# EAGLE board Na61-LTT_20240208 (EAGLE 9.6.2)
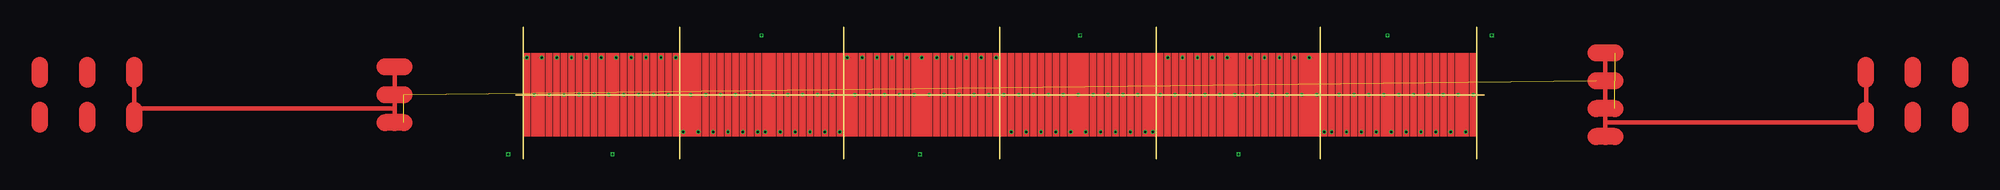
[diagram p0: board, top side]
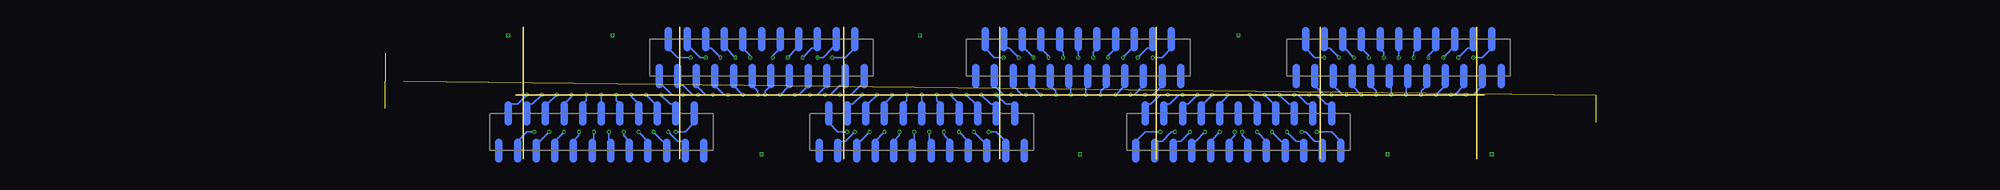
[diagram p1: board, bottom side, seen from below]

Size 104 x 14.2 mm. Coordinates in mm from the lower left corner, seen from the top.
Outline: 52,0 52,14.2
Outline: 35.2,0 35.2,14.2
Outline: 17.6,0 17.6,14.2
Outline: 0.8,0 0.8,14.2
Outline: 68.8,0 68.8,14.2
Outline: 86.4,0 86.4,14.2
Outline: 103.2,0 103.2,14.2
Outline: 0,6.9 104,6.9
Copper layers (1*16): Top 0.035mm / dielectric 1.5mm / Bottom 0.035mm
Design rules "default *": minimum track width 6mil, minimum drill 0.2mm, track to track 6mil, track to pad 6mil, pad to pad 6mil, via to via 6mil, smd to smd 6mil, copper to edge 40mil, drill to drill 6mil, minimum pad ring 8mil, minimum via ring 4mil, stop-mask expansion 4mil, vias tented up to drill 0mil, thermal gap 10mil

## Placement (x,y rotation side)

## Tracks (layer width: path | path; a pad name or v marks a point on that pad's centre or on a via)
S$1
  Bottom 0.8: 63.4,1.8 63.4,0
S$2
  Bottom 0.8: 62.4,4 62.4,5.8
S$3
  Bottom 0.8: 59.4,1.8 59.4,0
S$4
  Bottom 0.8: 56.4,4 56.4,5.8
S$5
  Bottom 0.8: 53.4,1.8 53.4,0
S$6
  Bottom 0.8: 52.4,4 52.4,5.8
S$7
  Bottom 0.8: 49.4,1.8 49.4,0
S$8
  Bottom 0.8: 50.4,4 50.4,5.8
S$9
  Bottom 0.8: 71.4,1.8 71.4,0
S$10
  Bottom 0.8: 70.4,4 70.4,5.8
S$11
  Bottom 0.8: 67.4,1.8 67.4,0
S$12
  Bottom 0.8: 66.4,4 66.4,5.8
S$13
  Bottom 0.8: 68.4,4 68.4,5.8
S$14
  Bottom 0.8: 69.4,1.8 69.4,0
S$15
  Bottom 0.8: 65.4,1.8 65.4,0
S$16
  Bottom 0.8: 64.4,4 64.4,5.8
S$17
  Bottom 0.8: 60.4,4 60.4,5.8
S$18
  Bottom 0.8: 61.4,1.8 61.4,0
S$19
  Bottom 0.8: 57.4,1.8 57.4,0
S$20
  Bottom 0.8: 58.4,4 58.4,5.8
S$21
  Bottom 0.8: 54.4,4 54.4,5.8
S$22
  Bottom 0.8: 55.4,1.8 55.4,0
S$23
  Bottom 0.8: 51.4,1.8 51.4,0
S$24
  Bottom 0.8: 44.6,9.8 44.6,8
S$25
  Bottom 0.8: 46.6,9.8 46.6,8
S$26
  Bottom 0.8: 43.6,12 43.6,13.8
S$27
  Bottom 0.8: 45.6,12 45.6,13.8
S$28
  Bottom 0.8: 40.6,9.8 40.6,8
S$29
  Bottom 0.8: 42.6,9.8 42.6,8
S$30
  Bottom 0.8: 41.6,12 41.6,13.8
S$31
  Bottom 0.8: 39.6,12 39.6,13.8
S$32
  Bottom 0.8: 38.6,9.8 38.6,8
S$33
  Bottom 0.8: 36.6,9.8 36.6,8
S$34
  Bottom 0.8: 37.6,12 37.6,13.8
S$35
  Bottom 0.8: 35.6,12 35.6,13.8
S$36
  Bottom 0.8: 34.6,9.8 34.6,8
S$37
  Bottom 0.8: 32.6,9.8 32.6,8
S$38
  Bottom 0.8: 33.6,12 33.6,13.8
S$39
  Bottom 0.8: 52.6,9.8 52.6,8
S$40
  Bottom 0.8: 54.6,9.8 54.6,8
S$41
  Bottom 0.8: 51.6,12 51.6,13.8
S$42
  Bottom 0.8: 53.6,12 53.6,13.8
S$43
  Bottom 0.8: 48.6,9.8 48.6,8
S$44
  Bottom 0.8: 50.6,9.8 50.6,8
S$45
  Bottom 0.8: 47.6,12 47.6,13.8
S$46
  Bottom 0.8: 49.6,12 49.6,13.8
S$47
  Bottom 0.8: 27.4,1.8 27.4,0
S$48
  Bottom 0.8: 29.4,1.8 29.4,0
S$49
  Bottom 0.8: 26.4,4 26.4,5.8
S$50
  Bottom 0.8: 28.4,4 28.4,5.8
S$51
  Bottom 0.8: 23.4,1.8 23.4,0
S$52
  Bottom 0.8: 25.4,1.8 25.4,0
S$53
  Bottom 0.8: 24.4,4 24.4,5.8
S$54
  Bottom 0.8: 22.4,4 22.4,5.8
S$55
  Bottom 0.8: 21.4,1.8 21.4,0
S$56
  Bottom 0.8: 19.4,1.8 19.4,0
S$57
  Bottom 0.8: 20.4,4 20.4,5.8
S$58
  Bottom 0.8: 18.4,4 18.4,5.8
S$59
  Bottom 0.8: 17.4,1.8 17.4,0
S$60
  Bottom 0.8: 15.4,1.8 15.4,0
S$61
  Bottom 0.8: 16.4,4 16.4,5.8
S$62
  Bottom 0.8: 35.4,1.8 35.4,0
S$63
  Bottom 0.8: 37.4,1.8 37.4,0
S$64
  Bottom 0.8: 34.4,4 34.4,5.8
S$65
  Bottom 0.8: 36.4,4 36.4,5.8
S$66
  Bottom 0.8: 31.4,1.8 31.4,0
S$67
  Bottom 0.8: 33.4,1.8 33.4,0
S$68
  Bottom 0.8: 30.4,4 30.4,5.8
S$69
  Bottom 0.8: 32.4,4 32.4,5.8
S$70
  Bottom 0.8: 78.6,9.8 78.6,8
S$71
  Bottom 0.8: 80.6,9.8 80.6,8
S$72
  Bottom 0.8: 77.6,12 77.6,13.8
S$73
  Bottom 0.8: 79.6,12 79.6,13.8
S$74
  Bottom 0.8: 74.6,9.8 74.6,8
S$75
  Bottom 0.8: 76.6,9.8 76.6,8
S$76
  Bottom 0.8: 75.6,12 75.6,13.8
S$77
  Bottom 0.8: 73.6,12 73.6,13.8
S$78
  Bottom 0.8: 72.6,9.8 72.6,8
S$79
  Bottom 0.8: 70.6,9.8 70.6,8
S$80
  Bottom 0.8: 71.6,12 71.6,13.8
S$81
  Bottom 0.8: 69.6,12 69.6,13.8
S$82
  Bottom 0.8: 68.6,9.8 68.6,8
S$83
  Bottom 0.8: 66.6,9.8 66.6,8
S$84
  Bottom 0.8: 67.6,12 67.6,13.8
S$85
  Bottom 0.8: 86.6,9.8 86.6,8
S$86
  Bottom 0.8: 88.6,9.8 88.6,8
S$87
  Bottom 0.8: 85.6,12 85.6,13.8
S$88
  Bottom 0.8: 87.6,12 87.6,13.8
S$89
  Bottom 0.8: 82.6,9.8 82.6,8
S$90
  Bottom 0.8: 84.6,9.8 84.6,8
S$91
  Bottom 0.8: 81.6,12 81.6,13.8
S$92
  Bottom 0.8: 83.6,12 83.6,13.8
S$93
  Bottom 0.8: 10.2,9.8 10.2,8
S$94
  Bottom 0.8: 12.2,9.8 12.2,8
S$95
  Bottom 0.8: 9.2,12 9.2,13.8
S$96
  Bottom 0.8: 11.2,12 11.2,13.8
S$97
  Bottom 0.8: 6.2,9.8 6.2,8
S$98
  Bottom 0.8: 8.2,9.8 8.2,8
S$99
  Bottom 0.8: 7.2,12 7.2,13.8
S$100
  Bottom 0.8: 5.2,12 5.2,13.8
S$101
  Bottom 0.8: 4.2,9.8 4.2,8
S$102
  Bottom 0.8: 2.2,9.8 2.2,8
S$103
  Bottom 0.8: 3.2,12 3.2,13.8
S$104
  Bottom 0.8: 1.2,12 1.2,13.8
S$105
  Bottom 0.8: 0.2,9.8 0.2,8
S$106
  Bottom 0.8: -1.8,9.8 -1.8,8
S$107
  Bottom 0.8: -0.8,12 -0.8,13.8
S$108
  Bottom 0.8: 18.2,9.8 18.2,8
S$109
  Bottom 0.8: 20.2,9.8 20.2,8
S$110
  Bottom 0.8: 17.2,12 17.2,13.8
S$111
  Bottom 0.8: 19.2,12 19.2,13.8
S$112
  Bottom 0.8: 14.2,9.8 14.2,8
S$113
  Bottom 0.8: 16.2,9.8 16.2,8
S$114
  Bottom 0.8: 13.2,12 13.2,13.8
S$115
  Bottom 0.8: 15.2,12 15.2,13.8
S$116
  Bottom 0.8: 95.8,1.8 95.8,0
S$117
  Bottom 0.8: 97.8,1.8 97.8,0
S$118
  Bottom 0.8: 94.8,4 94.8,5.8
S$119
  Bottom 0.8: 96.8,4 96.8,5.8
S$120
  Bottom 0.8: 91.8,1.8 91.8,0
S$121
  Bottom 0.8: 93.8,1.8 93.8,0
S$122
  Bottom 0.8: 92.8,4 92.8,5.8
S$123
  Bottom 0.8: 90.8,4 90.8,5.8
S$124
  Bottom 0.8: 89.8,1.8 89.8,0
S$125
  Bottom 0.8: 87.8,1.8 87.8,0
S$126
  Bottom 0.8: 88.8,4 88.8,5.8
S$127
  Bottom 0.8: 86.8,4 86.8,5.8
S$128
  Bottom 0.8: 85.8,1.8 85.8,0
S$129
  Bottom 0.8: 83.8,1.8 83.8,0
S$130
  Bottom 0.8: 84.8,4 84.8,5.8
S$131
  Bottom 0.8: 103.8,1.8 103.8,0
S$132
  Bottom 0.8: 105.8,1.8 105.8,0
S$133
  Bottom 0.8: 102.8,4 102.8,5.8
S$134
  Bottom 0.8: 104.8,4 104.8,5.8
S$135
  Bottom 0.8: 99.8,1.8 99.8,0
S$136
  Bottom 0.8: 101.8,1.8 101.8,0
S$137
  Bottom 0.8: 98.8,4 98.8,5.8
S$138
  Bottom 0.8: 100.8,4 100.8,5.8
S$139  (4 unrouted)
  Top 0.508: -13,9.9 -13,5.4 | -13,5.4 -13,3.9 | -13,5.4 -40.92,5.4 -40.92,7.9 | 117,11.4 117,3.9 | 117,3.9 117,2.4 | 117,3.9 145,3.9 145,8.9
  Top 1.8: -12,6.9 -14,6.9 | -12,9.9 -13,9.9 -14,9.9 | -12,3.9 -13,3.9 -14,3.9 | 118,8.4 116,8.4 | 118,11.4 117,11.4 116,11.4 | 118,5.4 116,5.4 | 118,2.4 117,2.4 116,2.4
S$140
  Top 1.778: -51.08,8.55 -51.08,10.07
S$141  (via drill 0.2)
  other vias: 26.4,13.3
S$142
  Top 1.778: -46,8.55 -46,10.07
S$143
  Top 1.778: -40.92,8.55 -40.92,10.07
S$144
  Top 1.778: 144.92,3.73 144.92,5.25
S$146
  Top 1.778: 144.92,8.55 144.92,10.07
S$147
  Top 1.778: 150,3.73 150,5.25
S$148
  Top 1.778: 150,8.55 150,10.07
S$149
  Top 1.778: 155.08,3.73 155.08,5.25
S$150
  Top 1.778: 155.08,8.55 155.08,10.07
S$151  (via drill 0.2)
  other vias: 43.4,0.5
S$152  (via drill 0.2)
  other vias: 60.6,13.3
S$153  (via drill 0.2)
  other vias: 77.6,0.5
S$154  (via drill 0.2)
  other vias: 93.6,13.3
S$155  (via drill 0.2)
  other vias: 104.8,13.3
S$156  (via drill 0.2)
  other vias: 10.4,0.5
S$157  (via drill 0.2)
  other vias: -0.8,0.5
S$162  (via drill 0.2)
  other vias: 1.2,10.9
S$163  (via drill 0.2)
  other vias: 2.8,10.9
S$164  (via drill 0.2)
  other vias: 4.4,10.9
S$165  (via drill 0.2)
  other vias: 6,10.9
S$166  (via drill 0.2)
  other vias: 7.6,10.9
S$167  (via drill 0.2)
  other vias: 9.2,10.9
S$168  (via drill 0.2)
  other vias: 10.8,10.9
S$169  (via drill 0.2)
  other vias: 12.4,10.9
S$170  (via drill 0.2)
  other vias: 14,10.9
S$171  (via drill 0.2)
  other vias: 15.6,10.9
S$172  (via drill 0.2)
  other vias: 17.2,10.9
S$173  (via drill 0.2)
  other vias: 2,6.9
S$174  (via drill 0.2)
  other vias: 3.6,6.9
S$175  (via drill 0.2)
  other vias: 5.2,6.9
S$176  (via drill 0.2)
  other vias: 6.8,6.9
S$177  (via drill 0.2)
  other vias: 8.4,6.9
S$178  (via drill 0.2)
  other vias: 10,6.9
S$179  (via drill 0.2)
  other vias: 11.6,6.9
S$180  (via drill 0.2)
  other vias: 13.2,6.9
S$181  (via drill 0.2)
  other vias: 14.8,6.9
S$182  (via drill 0.2)
  other vias: 16.4,6.9
S$183  (via drill 0.2)
  other vias: 18,2.9
S$184  (via drill 0.2)
  other vias: 19.6,2.9
S$185  (via drill 0.2)
  other vias: 21.2,2.9
S$186  (via drill 0.2)
  other vias: 22.8,2.9
S$187  (via drill 0.2)
  other vias: 24.4,2.9
S$188  (via drill 0.2)
  other vias: 18.8,6.9
S$189  (via drill 0.2)
  other vias: 20.4,6.9
S$190  (via drill 0.2)
  other vias: 22,6.9
S$191  (via drill 0.2)
  other vias: 23.6,6.9
S$192  (via drill 0.2)
  other vias: 25.2,6.9
S$193  (via drill 0.2)
  other vias: 26,2.9
S$194  (via drill 0.2)
  other vias: 51.6,10.9
S$195  (via drill 0.2)
  other vias: 50,10.9
S$196  (via drill 0.2)
  other vias: 48.4,10.9
S$197  (via drill 0.2)
  other vias: 46.8,10.9
S$198  (via drill 0.2)
  other vias: 45.2,10.9
S$199  (via drill 0.2)
  other vias: 43.6,10.9
S$200  (via drill 0.2)
  other vias: 42,10.9
S$201  (via drill 0.2)
  other vias: 40.4,10.9
S$202  (via drill 0.2)
  other vias: 38.8,10.9
S$203  (via drill 0.2)
  other vias: 37.2,10.9
S$204  (via drill 0.2)
  other vias: 35.6,10.9
S$205  (via drill 0.2)
  other vias: 50.8,6.9
S$206  (via drill 0.2)
  other vias: 49.2,6.9
S$207  (via drill 0.2)
  other vias: 47.6,6.9
S$208  (via drill 0.2)
  other vias: 46,6.9
S$209  (via drill 0.2)
  other vias: 44.4,6.9
S$210  (via drill 0.2)
  other vias: 42.8,6.9
S$211  (via drill 0.2)
  other vias: 41.2,6.9
S$212  (via drill 0.2)
  other vias: 39.6,6.9
S$213  (via drill 0.2)
  other vias: 38,6.9
S$214  (via drill 0.2)
  other vias: 36.4,6.9
S$215  (via drill 0.2)
  other vias: 34.8,2.9
S$216  (via drill 0.2)
  other vias: 33.2,2.9
S$217  (via drill 0.2)
  other vias: 31.6,2.9
S$218  (via drill 0.2)
  other vias: 30,2.9
S$219  (via drill 0.2)
  other vias: 28.4,2.9
S$220  (via drill 0.2)
  other vias: 34,6.9
S$221  (via drill 0.2)
  other vias: 32.4,6.9
S$222  (via drill 0.2)
  other vias: 30.8,6.9
S$223  (via drill 0.2)
  other vias: 29.2,6.9
S$224  (via drill 0.2)
  other vias: 27.6,6.9
S$225  (via drill 0.2)
  other vias: 26.8,2.9
S$226  (via drill 0.2)
  other vias: 52.4,6.9
S$227  (via drill 0.2)
  other vias: 54,6.9
S$228  (via drill 0.2)
  other vias: 55.6,6.9
S$229  (via drill 0.2)
  other vias: 57.2,6.9
S$230  (via drill 0.2)
  other vias: 58.8,6.9
S$231  (via drill 0.2)
  other vias: 60.4,6.9
S$232  (via drill 0.2)
  other vias: 62,6.9
S$233  (via drill 0.2)
  other vias: 63.6,6.9
S$234  (via drill 0.2)
  other vias: 65.2,6.9
S$235  (via drill 0.2)
  other vias: 66.8,6.9
S$236  (via drill 0.2)
  other vias: 68.4,2.9
S$237  (via drill 0.2)
  other vias: 53.2,2.9
S$238  (via drill 0.2)
  other vias: 54.8,2.9
S$239  (via drill 0.2)
  other vias: 56.4,2.9
S$240  (via drill 0.2)
  other vias: 58,2.9
S$241  (via drill 0.2)
  other vias: 59.6,2.9
S$242  (via drill 0.2)
  other vias: 61.2,2.9
S$243  (via drill 0.2)
  other vias: 62.8,2.9
S$244  (via drill 0.2)
  other vias: 64.4,2.9
S$245  (via drill 0.2)
  other vias: 66,2.9
S$246  (via drill 0.2)
  other vias: 67.6,2.9
S$247  (via drill 0.2)
  other vias: 69.2,6.9
S$248  (via drill 0.2)
  other vias: 70.8,6.9
S$249  (via drill 0.2)
  other vias: 72.4,6.9
S$250  (via drill 0.2)
  other vias: 70,10.9
S$251  (via drill 0.2)
  other vias: 71.6,10.9
S$252  (via drill 0.2)
  other vias: 73.2,10.9
S$253  (via drill 0.2)
  other vias: 74,6.9
S$254  (via drill 0.2)
  other vias: 74.8,10.9
S$255  (via drill 0.2)
  other vias: 75.6,6.9
S$256  (via drill 0.2)
  other vias: 76.4,10.9
S$257  (via drill 0.2)
  other vias: 77.2,6.9
S$258  (via drill 0.2)
  other vias: 102.8,6.9
S$259  (via drill 0.2)
  other vias: 101.2,6.9
S$260  (via drill 0.2)
  other vias: 99.6,6.9
S$261  (via drill 0.2)
  other vias: 98,6.9
S$262  (via drill 0.2)
  other vias: 96.4,6.9
S$263  (via drill 0.2)
  other vias: 94.8,6.9
S$264  (via drill 0.2)
  other vias: 93.2,6.9
S$265  (via drill 0.2)
  other vias: 91.6,6.9
S$266  (via drill 0.2)
  other vias: 90,6.9
S$267  (via drill 0.2)
  other vias: 88.4,6.9
S$268  (via drill 0.2)
  other vias: 86.8,2.9
S$269  (via drill 0.2)
  other vias: 102,2.9
S$270  (via drill 0.2)
  other vias: 100.4,2.9
S$271  (via drill 0.2)
  other vias: 98.8,2.9
S$272  (via drill 0.2)
  other vias: 97.2,2.9
S$273  (via drill 0.2)
  other vias: 95.6,2.9
S$274  (via drill 0.2)
  other vias: 94,2.9
S$275  (via drill 0.2)
  other vias: 92.4,2.9
S$276  (via drill 0.2)
  other vias: 90.8,2.9
S$277  (via drill 0.2)
  other vias: 89.2,2.9
S$278  (via drill 0.2)
  other vias: 87.6,2.9
S$279  (via drill 0.2)
  other vias: 86,6.9
S$280  (via drill 0.2)
  other vias: 84.4,6.9
S$281  (via drill 0.2)
  other vias: 82.8,6.9
S$282  (via drill 0.2)
  other vias: 85.2,10.9
S$283  (via drill 0.2)
  other vias: 83.6,10.9
S$284  (via drill 0.2)
  other vias: 82,10.9
S$285  (via drill 0.2)
  other vias: 81.2,6.9
S$286  (via drill 0.2)
  other vias: 80.4,10.9
S$287  (via drill 0.2)
  other vias: 79.6,6.9
S$288  (via drill 0.2)
  other vias: 78.8,10.9
S$289  (via drill 0.2)
  other vias: 78,6.9
S$290
  Bottom 0.152: -0.8,11.9 0.2,10.9
S$291
  Bottom 0.152: 0.2,10.9 1.2,10.9
S$292
  Bottom 0.152: 1.2,11.9 1.8,11.9
S$293
  Bottom 0.152: 1.8,11.9 2.8,10.9
S$294
  Bottom 0.152: 3.2,11.9 3.4,11.9
S$295
  Bottom 0.152: 3.4,11.9 4.4,10.9
S$296
  Bottom 0.152: 5.2,11.9 6,11.1
S$297
  Bottom 0.152: 6,11.1 6,10.9
S$298
  Bottom 0.152: 7.2,11.9 7.6,11.5
S$299
  Bottom 0.152: 7.6,11.5 7.6,10.9
S$300
  Bottom 0.152: 9.2,11.9 9.2,10.9
S$301
  Bottom 0.152: 11.2,11.9 10.8,11.5
S$302
  Bottom 0.152: 10.8,11.5 10.8,10.9
S$303
  Bottom 0.152: 13.2,11.9 12.4,11.1
S$304
  Bottom 0.152: 12.4,11.1 12.4,10.9
S$305
  Bottom 0.152: 15.2,11.9 15,11.9
S$306
  Bottom 0.152: 15,11.9 14,10.9
S$307
  Bottom 0.152: 17.2,11.9 16.6,11.9
S$308
  Bottom 0.152: 16.6,11.9 15.6,10.9
S$309
  Bottom 0.152: 19.2,11.9 18.2,10.9
S$310
  Bottom 0.152: 18.2,10.9 17.2,10.9
S$311
  Bottom 0.152: 0.2,7.9 1.2,6.9
S$312
  Bottom 0.152: 1.2,6.9 2,6.9
S$313
  Bottom 0.152: 2.2,7.9 3.2,6.9
S$314
  Bottom 0.152: 3.2,6.9 3.6,6.9
S$315
  Bottom 0.152: 4.2,7.9 5.2,6.9
S$316
  Bottom 0.152: 6.2,7.9 6.8,7.3
S$317
  Bottom 0.152: 6.8,7.3 6.8,6.9
S$318
  Bottom 0.152: 8.2,7.9 8.4,7.7
S$319
  Bottom 0.152: 8.4,7.7 8.4,6.9
S$320
  Bottom 0.152: 10.2,7.9 10,7.7
S$321
  Bottom 0.152: 10,7.7 10,6.9
S$322
  Bottom 0.152: 12.2,7.9 11.6,7.3
S$323
  Bottom 0.152: 11.6,7.3 11.6,6.9
S$324
  Bottom 0.152: 14.2,7.9 13.2,6.9
S$325
  Bottom 0.152: 16.2,7.9 15.2,6.9
S$326
  Bottom 0.152: 15.2,6.9 14.8,6.9
S$327
  Bottom 0.152: 18.2,7.9 17.2,6.9
S$328
  Bottom 0.152: 17.2,6.9 16.4,6.9
S$329
  Bottom 0.152: 15.4,1.9 16.4,2.9
S$330
  Bottom 0.152: 16.4,2.9 18,2.9
S$331
  Bottom 0.152: 17.4,1.9 18.2,1.9
S$332
  Bottom 0.152: 18.2,1.9 19.2,2.9
S$333
  Bottom 0.152: 19.2,2.9 19.6,2.9
S$334
  Bottom 0.152: 19.4,1.9 20.2,1.9
S$335
  Bottom 0.152: 20.2,1.9 21.2,2.9
S$336
  Bottom 0.152: 21.4,1.9 21.8,1.9
S$337
  Bottom 0.152: 21.8,1.9 22.8,2.9
S$338
  Bottom 0.152: 23.4,1.9 24.4,2.9
S$339
  Bottom 0.152: 25.4,1.9 26,2.5
S$340
  Bottom 0.152: 26,2.5 26,2.9
S$341
  Bottom 0.152: 16.4,5.9 17,5.9
S$342
  Bottom 0.152: 17,5.9 18,6.9
S$343
  Bottom 0.152: 18,6.9 18.8,6.9
S$344
  Bottom 0.152: 18.4,5.9 19,5.9
S$345
  Bottom 0.152: 19,5.9 20,6.9
S$346
  Bottom 0.152: 20,6.9 20.4,6.9
S$347
  Bottom 0.152: 20.4,5.9 21,5.9
S$348
  Bottom 0.152: 21,5.9 22,6.9
S$349
  Bottom 0.152: 22.4,5.9 22.6,5.9
S$350
  Bottom 0.152: 22.6,5.9 23.6,6.9
S$351
  Bottom 0.152: 24.4,5.9 25.2,6.7
S$352
  Bottom 0.152: 25.2,6.7 25.2,6.9
S$353
  Bottom 0.152: 53.6,11.9 52.6,10.9
S$354
  Bottom 0.152: 52.6,10.9 51.6,10.9
S$355
  Bottom 0.152: 51.6,11.9 51,11.9
S$356
  Bottom 0.152: 51,11.9 50,10.9
S$357
  Bottom 0.152: 49.6,11.9 49.4,11.9
S$358
  Bottom 0.152: 49.4,11.9 48.4,10.9
S$359
  Bottom 0.152: 47.6,11.9 46.8,11.1
S$360
  Bottom 0.152: 46.8,11.1 46.8,10.9
S$361
  Bottom 0.152: 45.6,11.9 45.2,11.5
S$362
  Bottom 0.152: 45.2,11.5 45.2,10.9
S$363
  Bottom 0.152: 43.6,11.9 43.6,10.9
S$364
  Bottom 0.152: 41.6,11.9 42,11.5
S$365
  Bottom 0.152: 42,11.5 42,10.9
S$366
  Bottom 0.152: 39.6,11.9 40.4,11.1
S$367
  Bottom 0.152: 40.4,11.1 40.4,10.9
S$368
  Bottom 0.152: 37.6,11.9 37.8,11.9
S$369
  Bottom 0.152: 37.8,11.9 38.8,10.9
S$370
  Bottom 0.152: 35.6,11.9 36.2,11.9
S$371
  Bottom 0.152: 36.2,11.9 37.2,10.9
S$372
  Bottom 0.152: 33.6,11.9 34.6,10.9
S$373
  Bottom 0.152: 34.6,10.9 35.6,10.9
S$374
  Bottom 0.152: 52.6,7.9 51.6,6.9
S$375
  Bottom 0.152: 51.6,6.9 50.8,6.9
S$376
  Bottom 0.152: 50.6,7.9 49.6,6.9
S$377
  Bottom 0.152: 49.6,6.9 49.2,6.9
S$378
  Bottom 0.152: 48.6,7.9 47.6,6.9
S$379
  Bottom 0.152: 46.6,7.9 46,7.3
S$380
  Bottom 0.152: 46,7.3 46,6.9
S$381
  Bottom 0.152: 44.6,7.9 44.4,7.7
S$382
  Bottom 0.152: 44.4,7.7 44.4,6.9
S$383
  Bottom 0.152: 42.6,7.9 42.8,7.7
S$384
  Bottom 0.152: 42.8,7.7 42.8,6.9
S$385
  Bottom 0.152: 40.6,7.9 41.2,7.3
S$386
  Bottom 0.152: 41.2,7.3 41.2,6.9
S$387
  Bottom 0.152: 38.6,7.9 39.6,6.9
S$388
  Bottom 0.152: 36.6,7.9 37.6,6.9
S$389
  Bottom 0.152: 37.6,6.9 38,6.9
S$390
  Bottom 0.152: 34.6,7.9 35.6,6.9
S$391
  Bottom 0.152: 35.6,6.9 36.4,6.9
S$392
  Bottom 0.152: 37.4,1.9 36.4,2.9
S$393
  Bottom 0.152: 36.4,2.9 34.8,2.9
S$394
  Bottom 0.152: 35.4,1.9 34.6,1.9
S$395
  Bottom 0.152: 34.6,1.9 33.6,2.9
S$396
  Bottom 0.152: 33.6,2.9 33.2,2.9
S$397
  Bottom 0.152: 33.4,1.9 32.6,1.9
S$398
  Bottom 0.152: 32.6,1.9 31.6,2.9
S$399
  Bottom 0.152: 31.4,1.9 31,1.9
S$400
  Bottom 0.152: 31,1.9 30,2.9
S$401
  Bottom 0.152: 29.4,1.9 28.4,2.9
S$402
  Bottom 0.152: 27.4,1.9 26.8,2.5
S$403
  Bottom 0.152: 26.8,2.5 26.8,2.9
S$404
  Bottom 0.152: 36.4,5.9 35.8,5.9
S$405
  Bottom 0.152: 35.8,5.9 34.8,6.9
S$406
  Bottom 0.152: 34.8,6.9 34,6.9
S$407
  Bottom 0.152: 34.4,5.9 33.8,5.9
S$408
  Bottom 0.152: 33.8,5.9 32.8,6.9
S$409
  Bottom 0.152: 32.8,6.9 32.4,6.9
S$410
  Bottom 0.152: 32.4,5.9 31.8,5.9
S$411
  Bottom 0.152: 31.8,5.9 30.8,6.9
S$412
  Bottom 0.152: 30.4,5.9 30.2,5.9
S$413
  Bottom 0.152: 30.2,5.9 29.2,6.9
S$414
  Bottom 0.152: 28.4,5.9 27.6,6.7
S$415
  Bottom 0.152: 27.6,6.7 27.6,6.9
S$416
  Bottom 0.152: 52.4,5.9 53,5.9
S$417
  Bottom 0.152: 53,5.9 54,6.9
S$418
  Bottom 0.152: 54.4,5.9 54.6,5.9
S$419
  Bottom 0.152: 54.6,5.9 55.6,6.9
S$420
  Bottom 0.152: 56.4,5.9 57.2,6.7
S$421
  Bottom 0.152: 57.2,6.7 57.2,6.9
S$422
  Bottom 0.152: 58.4,5.9 58.8,6.3
S$423
  Bottom 0.152: 58.8,6.3 58.8,6.9
S$424
  Bottom 0.152: 60.4,5.9 60.4,6.9
S$425
  Bottom 0.152: 50.4,5.9 51.4,5.9
S$426
  Bottom 0.152: 51.4,5.9 52.4,6.9
S$427
  Bottom 0.152: 51.4,1.9 52.4,2.9
S$428
  Bottom 0.152: 52.4,2.9 53.2,2.9
S$429
  Bottom 0.152: 53.4,1.9 53.8,1.9
S$430
  Bottom 0.152: 53.8,1.9 54.8,2.9
S$431
  Bottom 0.152: 55.4,1.9 56.4,2.9
S$432
  Bottom 0.152: 57.4,1.9 58,2.5
S$433
  Bottom 0.152: 58,2.5 58,2.9
S$434
  Bottom 0.152: 59.4,1.9 59.6,2.1
S$435
  Bottom 0.152: 59.6,2.1 59.6,2.9
S$436
  Bottom 0.152: 61.4,1.9 61.2,2.1
S$437
  Bottom 0.152: 61.2,2.1 61.2,2.9
S$438
  Bottom 0.152: 63.4,1.9 62.8,2.5
S$439
  Bottom 0.152: 62.8,2.5 62.8,2.9
S$440
  Bottom 0.152: 65.4,1.9 64.4,2.9
S$441
  Bottom 0.152: 67.4,1.9 67,1.9
S$442
  Bottom 0.152: 67,1.9 66,2.9
S$443
  Bottom 0.152: 69.4,1.9 68.6,1.9
S$444
  Bottom 0.152: 68.6,1.9 67.6,2.9
S$445
  Bottom 0.152: 62.4,5.9 62,6.3
S$446
  Bottom 0.152: 62,6.3 62,6.9
S$447
  Bottom 0.152: 64.4,5.9 63.6,6.7
S$448
  Bottom 0.152: 63.6,6.7 63.6,6.9
S$449
  Bottom 0.152: 66.4,5.9 66.2,5.9
S$450
  Bottom 0.152: 66.2,5.9 65.2,6.9
S$451
  Bottom 0.152: 68.4,5.9 67.8,5.9
S$452
  Bottom 0.152: 67.8,5.9 66.8,6.9
S$453
  Bottom 0.152: 70.4,3.9 69.4,2.9
S$454
  Bottom 0.152: 69.4,2.9 68.4,2.9
S$455
  Bottom 0.152: 68.6,7.9 69.2,7.9
S$456
  Bottom 0.152: 69.2,7.9 70.2,6.9
S$457
  Bottom 0.152: 70.2,6.9 70.8,6.9
S$458
  Bottom 0.152: 70.6,7.9 71.6,6.9
S$459
  Bottom 0.152: 71.6,6.9 72.4,6.9
S$460
  Bottom 0.152: 72.6,7.9 73.6,6.9
S$461
  Bottom 0.152: 73.6,6.9 74,6.9
S$462
  Bottom 0.152: 74.6,7.9 75.6,6.9
S$463
  Bottom 0.152: 76.6,7.9 77.2,7.3
S$464
  Bottom 0.152: 77.2,7.3 77.2,6.9
S$465
  Bottom 0.152: 67.6,11.9 68.6,10.9
S$466
  Bottom 0.152: 68.6,10.9 70,10.9
S$467
  Bottom 0.152: 69.6,11.9 70,11.9
S$468
  Bottom 0.152: 70,11.9 71,10.9
S$469
  Bottom 0.152: 71,10.9 71.6,10.9
S$470
  Bottom 0.152: 71.6,11.9 72.2,11.9
S$471
  Bottom 0.152: 72.2,11.9 73.2,10.9
S$472
  Bottom 0.152: 73.6,11.9 73.8,11.9
S$473
  Bottom 0.152: 73.8,11.9 74.8,10.9
S$474
  Bottom 0.152: 75.6,11.9 76.4,11.1
S$475
  Bottom 0.152: 76.4,11.1 76.4,10.9
S$476
  Bottom 0.152: 69.2,6.9 68,6.9
S$477
  Bottom 0.152: 68,6.9 67,7.9
S$478
  Bottom 0.152: 67,7.9 66.6,7.9
S$479
  Bottom 0.152: 102.8,5.9 102.2,5.9
S$480
  Bottom 0.152: 102.2,5.9 101.2,6.9
S$481
  Bottom 0.152: 100.8,5.9 100.6,5.9
S$482
  Bottom 0.152: 100.6,5.9 99.6,6.9
S$483
  Bottom 0.152: 98.8,5.9 98,6.7
S$484
  Bottom 0.152: 98,6.7 98,6.9
S$485
  Bottom 0.152: 96.8,5.9 96.4,6.3
S$486
  Bottom 0.152: 96.4,6.3 96.4,6.9
S$487
  Bottom 0.152: 94.8,5.9 94.8,6.9
S$488
  Bottom 0.152: 104.8,5.9 103.8,5.9
S$489
  Bottom 0.152: 103.8,5.9 102.8,6.9
S$490
  Bottom 0.152: 103.8,1.9 102.8,2.9
S$491
  Bottom 0.152: 102.8,2.9 102,2.9
S$492
  Bottom 0.152: 101.8,1.9 101.4,1.9
S$493
  Bottom 0.152: 101.4,1.9 100.4,2.9
S$494
  Bottom 0.152: 99.8,1.9 98.8,2.9
S$495
  Bottom 0.152: 97.8,1.9 97.2,2.5
S$496
  Bottom 0.152: 97.2,2.5 97.2,2.9
S$497
  Bottom 0.152: 95.8,1.9 95.6,2.1
S$498
  Bottom 0.152: 95.6,2.1 95.6,2.9
S$499
  Bottom 0.152: 93.8,1.9 94,2.1
S$500
  Bottom 0.152: 94,2.1 94,2.9
S$501
  Bottom 0.152: 91.8,1.9 92.4,2.5
S$502
  Bottom 0.152: 92.4,2.5 92.4,2.9
S$503
  Bottom 0.152: 89.8,1.9 90.8,2.9
S$504
  Bottom 0.152: 87.8,1.9 88.2,1.9
S$505
  Bottom 0.152: 88.2,1.9 89.2,2.9
S$506
  Bottom 0.152: 85.8,1.9 86.6,1.9
S$507
  Bottom 0.152: 86.6,1.9 87.6,2.9
S$508
  Bottom 0.152: 92.8,5.9 93.2,6.3
S$509
  Bottom 0.152: 93.2,6.3 93.2,6.9
S$510
  Bottom 0.152: 90.8,5.9 91.6,6.7
S$511
  Bottom 0.152: 91.6,6.7 91.6,6.9
S$512
  Bottom 0.152: 88.8,5.9 89,5.9
S$513
  Bottom 0.152: 89,5.9 90,6.9
S$514
  Bottom 0.152: 86.8,5.9 87.4,5.9
S$515
  Bottom 0.152: 87.4,5.9 88.4,6.9
S$516
  Bottom 0.152: 84.8,3.9 85.8,2.9
S$517
  Bottom 0.152: 85.8,2.9 86.8,2.9
S$518
  Bottom 0.152: 86.6,7.9 86,7.9
S$519
  Bottom 0.152: 86,7.9 85,6.9
S$520
  Bottom 0.152: 85,6.9 84.4,6.9
S$521
  Bottom 0.152: 84.6,7.9 83.6,6.9
S$522
  Bottom 0.152: 83.6,6.9 82.8,6.9
S$523
  Bottom 0.152: 82.6,7.9 81.6,6.9
S$524
  Bottom 0.152: 81.6,6.9 81.2,6.9
S$525
  Bottom 0.152: 80.6,7.9 79.6,6.9
S$526
  Bottom 0.152: 78.6,7.9 78,7.3
S$527
  Bottom 0.152: 78,7.3 78,6.9
S$528
  Bottom 0.152: 87.6,11.9 86.6,10.9
S$529
  Bottom 0.152: 86.6,10.9 85.2,10.9
S$530
  Bottom 0.152: 85.6,11.9 85.2,11.9
S$531
  Bottom 0.152: 85.2,11.9 84.2,10.9
S$532
  Bottom 0.152: 84.2,10.9 83.6,10.9
S$533
  Bottom 0.152: 83.6,11.9 83,11.9
S$534
  Bottom 0.152: 83,11.9 82,10.9
S$535
  Bottom 0.152: 81.6,11.9 81.4,11.9
S$536
  Bottom 0.152: 81.4,11.9 80.4,10.9
S$537
  Bottom 0.152: 79.6,11.9 78.8,11.1
S$538
  Bottom 0.152: 78.8,11.1 78.8,10.9
S$539
  Bottom 0.152: 86,6.9 87.2,6.9
S$540
  Bottom 0.152: 87.2,6.9 88.2,7.9
S$541
  Bottom 0.152: 88.2,7.9 88.6,7.9
S$991
  Top 1.778: -51.08,3.73 -51.08,5.25
S$992
  Top 1.778: -46,3.73 -46,5.25
S$993
  Top 1.778: -40.92,3.73 -40.92,5.25
(copper drawn outside any net)
  shapes: Top area x128

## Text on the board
Dimension: 00.0 / - 08.4 / 16.8 / - 25.6 / 34.4 / - 42.8 / 51.2
Contour: Pad: 0.8 x 9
